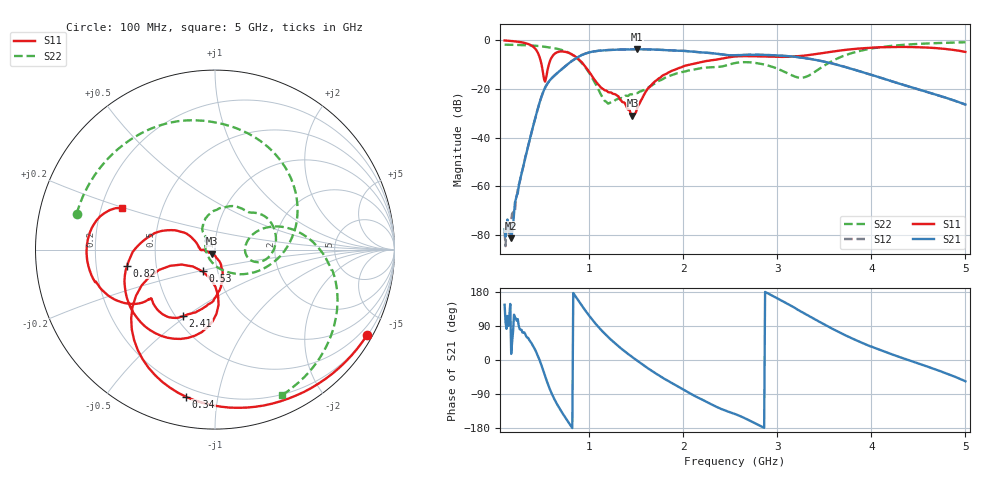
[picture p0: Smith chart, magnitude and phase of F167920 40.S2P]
!  2-Port S-parameters saved by WinCal
! VAR MeasName=S-Parameters (CALIBRATED_DATA) read from VNA (N5242A)
! VAR MeasDate=2016-11-22 9:57:23
! VAR NAME=F167920 40
! VAR FILENAME=F167920 40.S2P
! VAR DATE=2016-11-22 9:57:23
! VAR PHYS_PORTS=1,2
# Hz S DB R 50
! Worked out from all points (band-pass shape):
!   491 points, 100 MHz to 5 GHz, reference 50 ohm
!   highest |S21| = -3.84 dB at 1.51 GHz (marker M1); lowest = -81.2 dB at 170 MHz (marker M2)
!   |S21| within 3 dB of the highest: 889.7 MHz to 3.161 GHz (2.272 GHz wide, 112 % of centre)
!   lowest |S11| = -31.1 dB at 1.46 GHz (marker M3), VSWR 1.06, Z = 48.2 - j2.12 ohm
!   |S11| at or under -10 dB: 492 MHz to 571.7 MHz (79.76 MHz wide, 15 % of centre); 938 MHz to 2.086 GHz (1.148 GHz wide, 75.9 % of centre)
!   |S22| runs from -26.1 to -1.0 dB; largest |S21 - S12| = 0.0021
!   S11 on the Smith chart (normalised r, x): 100 MHz: 0.22, -3.82; 340 MHz: 0.15, -0.81; 530 MHz: 0.85, -0.21; 820 MHz: 0.34, -0.08; 2.41 GHz: 0.54, -0.49; 5 GHz: 0.29, +0.20
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1e8  -0.25 -29.3  -77.55 145.8  -78.60 76.3  -1.98 165.5
1.7e8  -0.47 -49.3  -81.20 16.0  -74.09 111.0  -2.03 155.2
3.4e8  -1.55 -101.1  -45.14 59.4  -45.02 61.3  -2.23 129.1
4.4e8  -4.39 -140.7  -30.01 18.6  -29.98 18.9  -2.45 111.8
5.3e8  -17.10 -119.7  -19.63 -41.9  -19.63 -41.9  -2.85 94.9
5.8e8  -8.92 -88.7  -16.60 -76.3  -16.60 -76.2  -3.13 85.0
6.5e8  -5.24 -114.7  -13.93 -113.2  -13.92 -113.1  -3.59 69.7
8.2e8  -6.07 -169.7  -8.55 -179.6  -8.53 -179.7  -6.09 22.4
9.2e8  -9.13 164.8  -6.21 144.2  -6.21 144.2  -9.47 -11.7
1.05e9  -16.01 151.6  -4.73 100.8  -4.73 100.8  -16.85 -60.6
1.19e9  -21.02 172.8  -4.18 63.2  -4.18 63.2  -25.70 -150.7
1.46e9  -31.06 -128.5  -3.88 7.3  -3.88 7.4  -22.22 127.3
1.51e9  -27.97 -83.1  -3.84 -1.9  -3.84 -1.9  -21.81 126.1
1.74e9  -15.77 -74.8  -4.07 -40.4  -4.06 -40.4  -16.83 118.8
2.03e9  -10.49 -94.8  -4.60 -82.5  -4.59 -82.5  -12.81 85.0
2.41e9  -7.70 -115.8  -5.98 -129.9  -5.96 -130.0  -10.89 46.3
2.55e9  -6.81 -124.4  -6.30 -142.4  -6.28 -142.5  -9.51 33.2
2.94e9  -6.94 -141.4  -6.27 170.6  -6.25 170.4  -10.96 -11.8
3.37e9  -6.07 -143.8  -7.95 111.5  -7.92 111.4  -13.82 18.8
3.71e9  -4.18 -152.9  -10.99 66.9  -10.96 66.6  -6.49 12.1
4.19e9  -2.95 -173.2  -16.63 17.5  -16.64 17.1  -2.56 -23.5
5e9  -4.94 156.0  -26.48 -56.1  -26.56 -56.2  -0.99 -65.2
